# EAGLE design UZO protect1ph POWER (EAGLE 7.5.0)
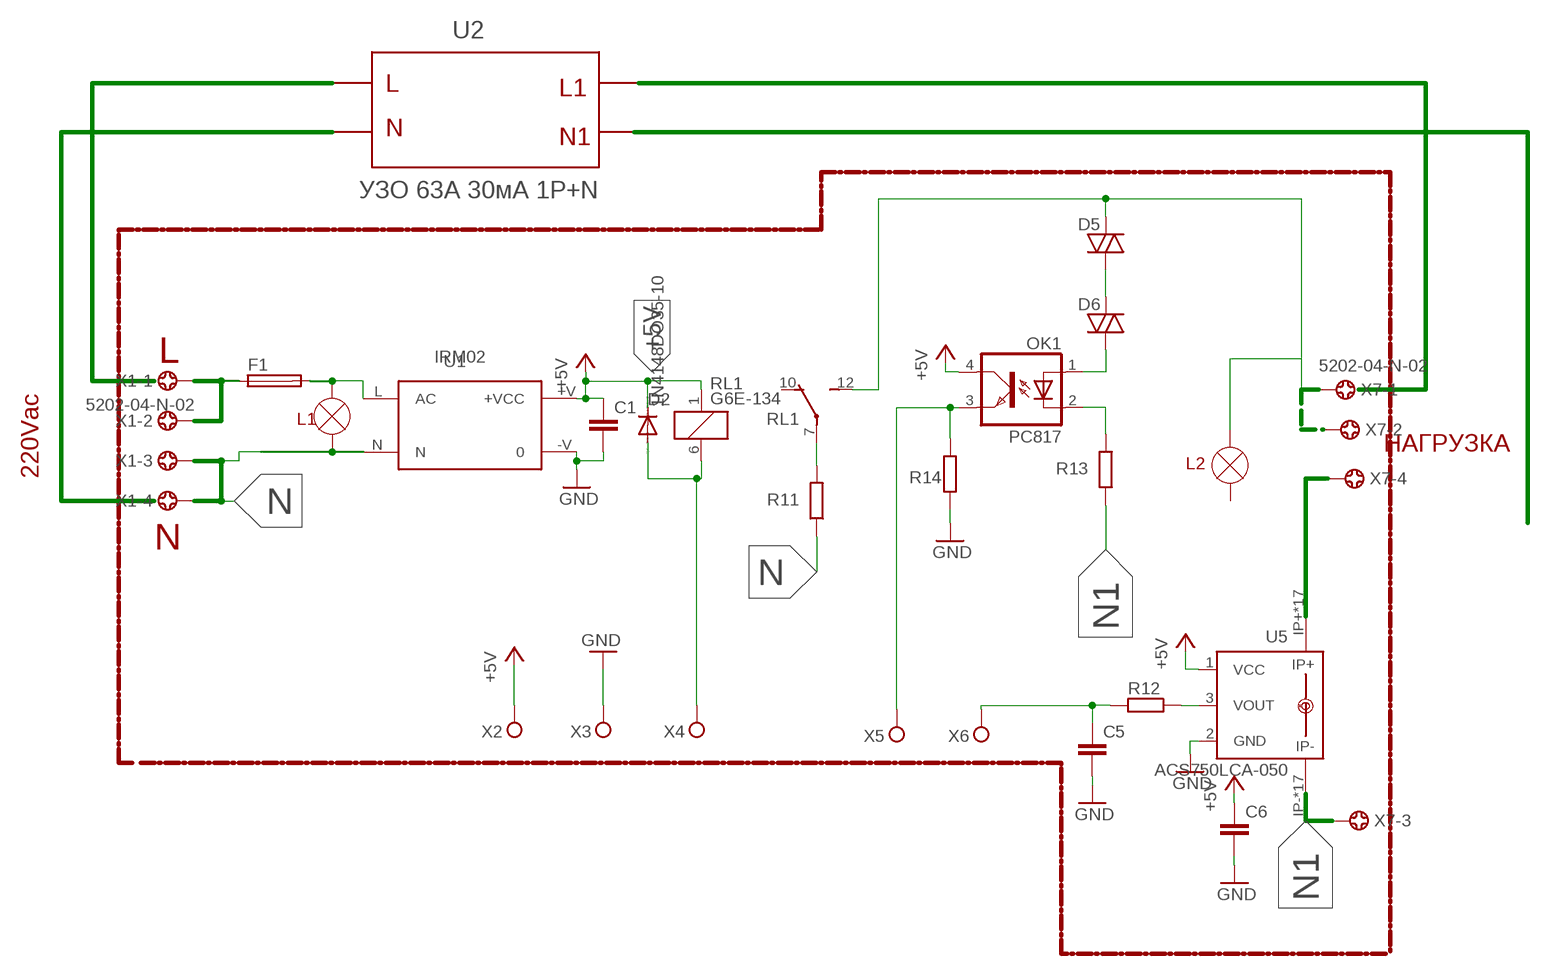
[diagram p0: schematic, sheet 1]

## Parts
C1  C-EUC1206  [C1206]
C5  C-EUC1206  [C1206]
C6  C-EUC1206  [C1206]
D2  1N4148DO35-10  [DO35-10]
D5  DIAC-DO35-10  [DO35-10]
D6  DIAC-DO35-10  [DO35-10]
F1  FUSEGSH15 1A 5x20mm  FUSEGSH15  [GSH15]
OK1  PC817  [DIL04]
R11  R-EU_0817/22  [P0817/22]
R12  R-EU_R1206  [R1206]
R13  R-EU_0817/22  [P0817/22]
R14  R-EU_R1206  [R1206]
RL1  G6E-134  [G6E]
U1  IRM02  [IRM02]
U5  ACS750LCA-050  [ACS75050]
X1  5202-04-N-02  [5202-04-N-02]
X2  TPPAD1-17  [P1-17]
X3  TPPAD1-17  [P1-17]
X4  TPPAD1-17  [P1-17]
X5  TPPAD1-17  [P1-17]
X6  TPPAD1-17  [P1-17]
X7  5202-04-N-02  [5202-04-N-02]

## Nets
+5V: C1.1 C6.1 D2.C OK1.4(COL) RL1.1 U1.+V(+VCC) U5.1(VCC) X2.TP
GND: C1.2 C5.2 C6.2 R14.1 U1.-V U5.2(GND) X3.TP
N: R11.1 U1.N X1.3 X1.4
N1: R13.1 U5.IP- U5.IP-@2(IP-) U5.IP-@3(IP-) U5.IP-@4(IP-) U5.IP-@5(IP-) U5.IP-@6(IP-) U5.IP-@7(IP-) U5.IP-@8(IP-) U5.IP-@9(IP-) U5.IP-@10(IP-) U5.IP-@11(IP-) U5.IP-@12(IP-) U5.IP-@13(IP-) U5.IP-@14(IP-) U5.IP-@15(IP-) U5.IP-@16(IP-) U5.IP-@17(IP-) X7.3
N$1: F1.1 X1.1 X1.2
N$2: R11.2 RL1.7(P)
N$3: F1.2 U1.L(AC)
N$4: D2.A RL1.6 X4.TP
N$5: U5.IP+ U5.IP+@2(IP+) U5.IP+@3(IP+) U5.IP+@4(IP+) U5.IP+@5(IP+) U5.IP+@6(IP+) U5.IP+@7(IP+) U5.IP+@8(IP+) U5.IP+@9(IP+) U5.IP+@10(IP+) U5.IP+@11(IP+) U5.IP+@12(IP+) U5.IP+@13(IP+) U5.IP+@14(IP+) U5.IP+@15(IP+) U5.IP+@16(IP+) U5.IP+@17(IP+) X7.4
N$8: D5.A D6.C
N$9: D6.A OK1.1(A)
N$10: OK1.2(C) R13.2
N$11: OK1.3(EMIT) R14.2 X5.TP
N$12: R12.1 U5.3(VOUT)
N$13: C5.1 R12.2 X6.TP
N$17: D5.C RL1.12(S) X7.1 X7.2
Unconnected: RL1.10(O)

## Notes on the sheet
- U2
- L | L1
- N
- N1
- УЗО 63А 30мА 1Р+N
- L
- L1
- НАГРУЗКА
- L2
- 220Vac
- N

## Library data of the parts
C1 C5 C6 = rcl:C-EU: CAPACITOR, European symbol
D2 = diode:1N4148: DIODE
D5 D6 = diode:DIAC-: DIAC
F1 = fuse:FUSE: Fuse; OC_FARNELL: unknown; OC_NEWARK: unknown
OK1 = optocoupler:PC817: SHARP OPTO COUPLER; MPN: PC817X4J000F; OC_FARNELL: 9707727; OC_NEWARK: 97K7059
R11-R14 = rcl:R-EU_: RESISTOR, European symbol
RL1 = relay:G6E-134
U1 = acdc:IRM02: 2W Single Output ACDC converter
U5 = allegro:ACS750*CA-050: Current Sensor display layer 49 Reference in BRD and place VIAs on circles Source: www.allegromicro.com/datafile/0750-050.pdf; MF: ALLEGRO MICROSYSTEMS, INC.; MPN: ACS750LCA-050; OC_FARNELL: 1457176; OC_NEWARK: 61H4464
X1 X7 = con-ebyelectro:5202-04-N-02: Barrier Blocks Sreies 5202 Source: http://www.ebyelectro.com/PDF/5202-XX-N-02.pdf; OC_FARNELL: unknown; OC_NEWARK: unknown
X2-X6 = testpad:TP: Test pad

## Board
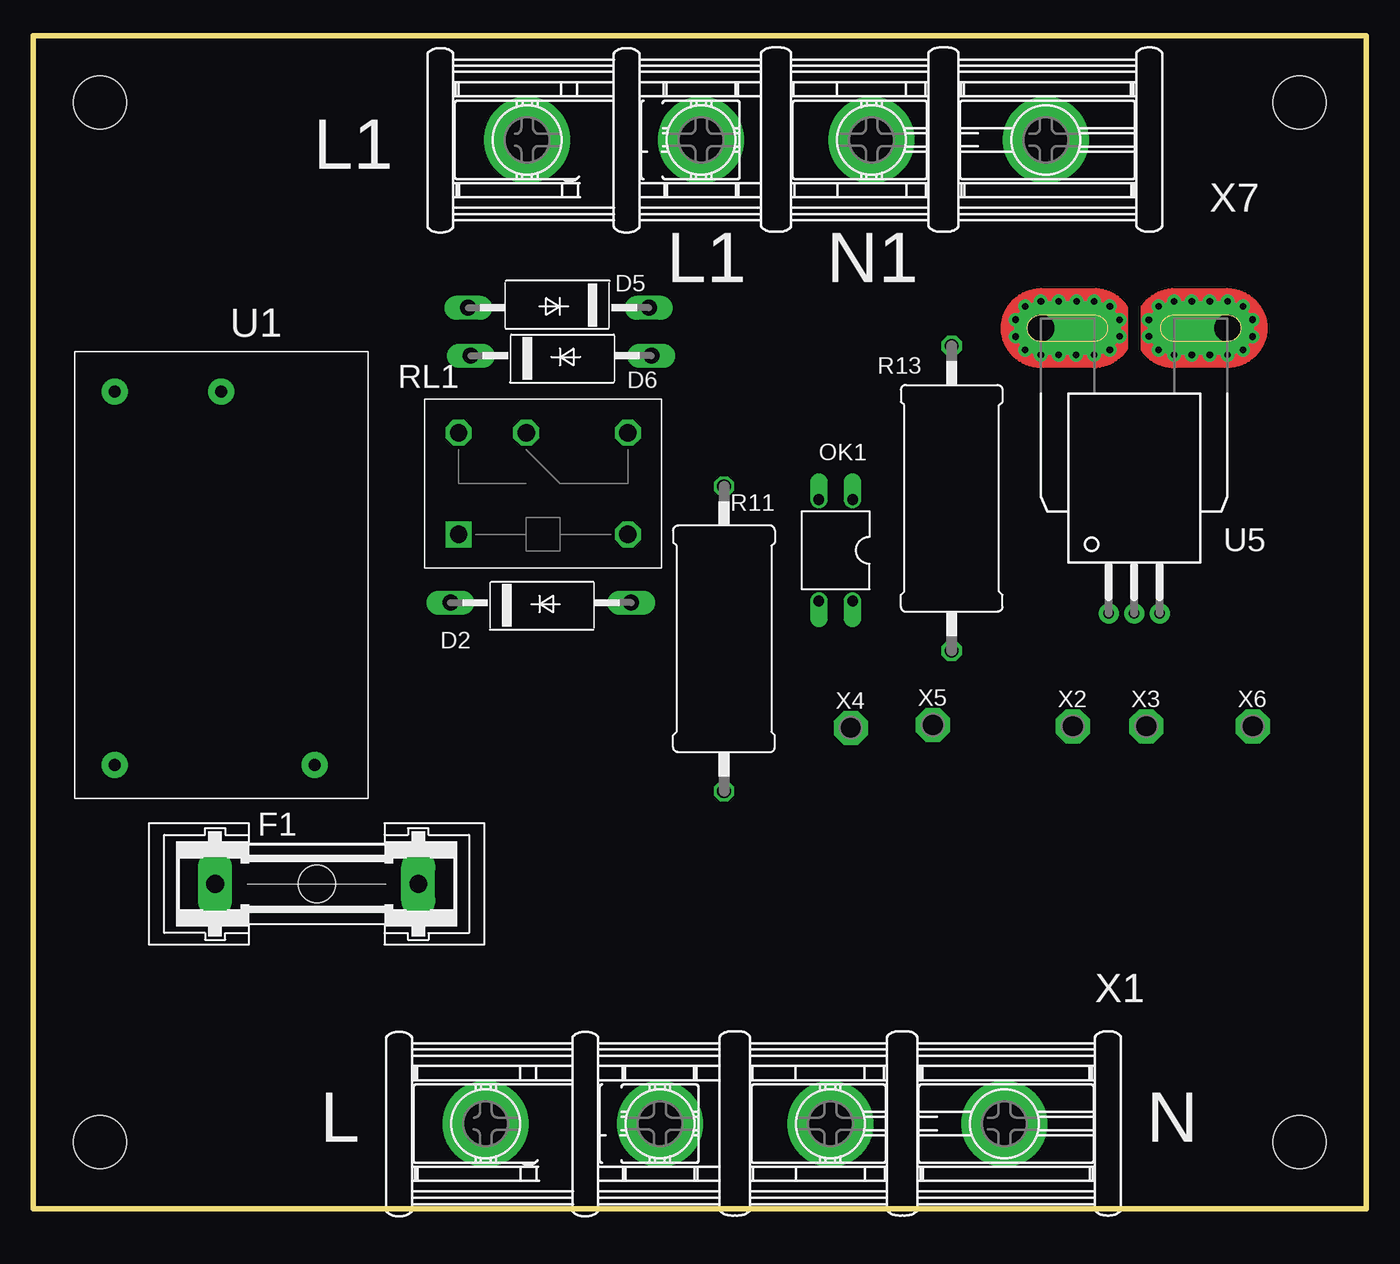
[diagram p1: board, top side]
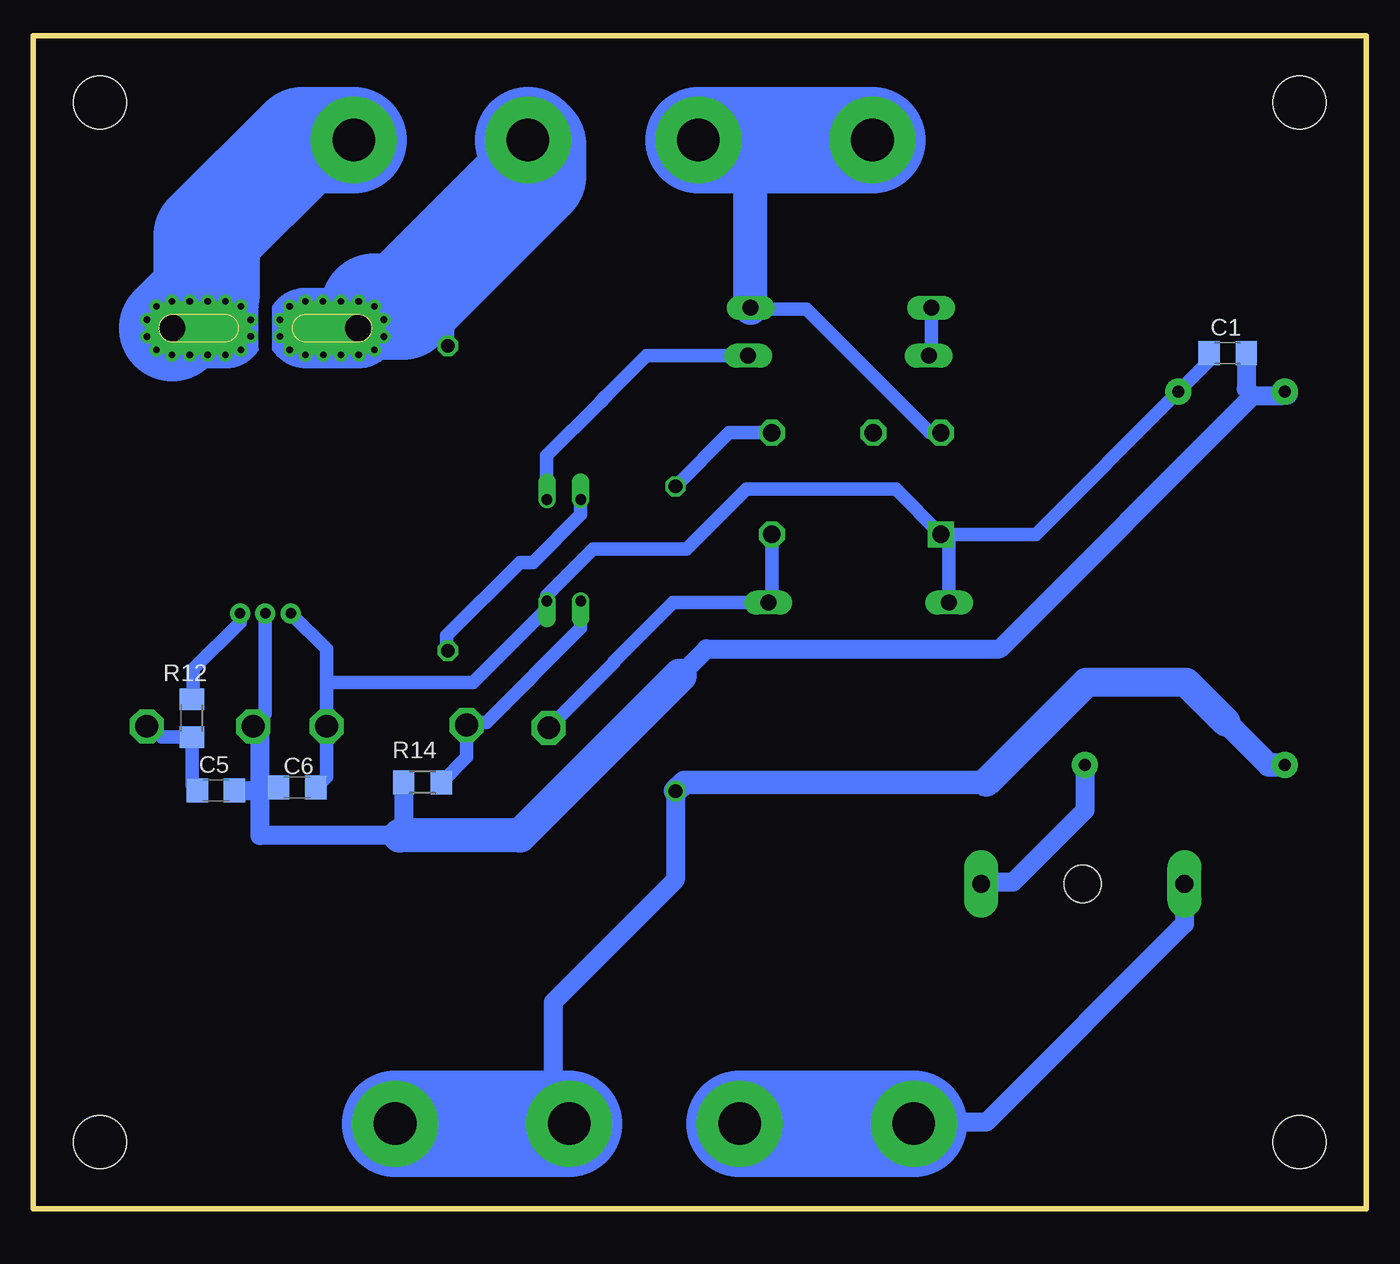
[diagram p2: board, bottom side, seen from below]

Size 100 x 88 mm. Coordinates in mm from the lower left corner, seen from the top.
Outline: 0,0 100,0 100,88 0,88 0,0
Copper layers (1*16): Top 0.035mm / dielectric 1.5mm / Bottom 0.035mm
Design rules "default *": minimum track width 10mil, minimum drill 10mil, track to track 8mil, track to pad 8mil, pad to pad 8mil, via to via 8mil, smd to smd 8mil, copper to edge 40mil, drill to drill 8mil, minimum pad ring 10mil, minimum via ring 8mil, stop-mask expansion 4mil, vias tented up to drill 0mil, thermal gap 10mil
Holes 4 mm at 5,5 95,5 95,83 5,83

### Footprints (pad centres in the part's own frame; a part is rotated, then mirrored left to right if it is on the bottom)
C1206 = smd 1.6 x 1.8: 1 -1.4,0; 2 1.4,0
DO35-10 = drill 1.2 long: A 8.18,0; C -5.38,0
GSH15 = drill 1.321 pad 2.54 long: 1 -7.62,0; 2 7.62,0 | hole 2.794: 0,0
DIL04 = drill 0.813 offset: 1 -1.27,-3.81; 2 1.27,-3.81; 3 1.27,3.81; 4 -1.27,3.81
P0817/22 = drill 1.016 octagon: 1 -11.43,0; 2 11.43,0
R1206 = smd 1.6 x 1.803: 1 -1.422,0; 2 1.422,0
G6E = drill 1.3 square: 1 0,0 | drill 1.3 octagon: 6 12.7,0; 7 12.7,7.62; 10 5.08,7.62; 12 0,7.62
IRM02 = drill 0.9 pad 1.93: +V 30.5,-11; -V 30.5,-3; L 2.5,-18; N 2.5,-3
ACS75050 = drill 0.8 pad 1.5: 1 -1.91,-21.4; 2 0,-21.4; 3 1.91,-21.4 | drill 2 pad 4 offset: IP+ 7,0; IP- -7,0 | drill 0.5 pad 0.9: IP+@2 8.89,-0.635; IP+@3 8.89,0.635; IP+@4 8.175,1.625; IP+@5 7,2; IP+@6 5.675,2; IP+@7 4.325,2; IP+@8 3,2; IP+@9 1.825,1.625; IP+@10 1.1,0.625; IP+@11 1.1,-0.625; IP+@12 1.825,-1.625; IP+@13 3,-2; IP+@14 4.325,-2; IP+@15 5.675,-2; IP+@16 7,-2; IP+@17 8.175,-1.625; IP-@2 -8.89,-0.635; IP-@3 -8.89,0.635; IP-@4 -8.175,1.625; IP-@5 -7,2; IP-@6 -5.675,2; IP-@7 -4.325,2; IP-@8 -3,2; IP-@9 -1.825,1.625; IP-@10 -1.1,0.625; IP-@11 -1.1,-0.625; IP-@12 -1.825,-1.625; IP-@13 -3,-2; IP-@14 -4.35,-2; IP-@15 -5.675,-2; IP-@16 -7,-2; IP-@17 -8.175,-1.625
5202-04-N-02 = drill 3.2 pad 6.452: 1 -14.875,0; 2 -1.815,0; 3 10.975,0; 4 24.035,0
P1-17 = drill 1.702 pad 2.54 octagon: TP 0,0

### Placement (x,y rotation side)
C1  10.4,64.21 0 bottom
C5  86.3,31.4 0 bottom
C6  80.2,31.6 180 bottom
D2  36.68,45.47 0 top
D5  40.8,67.6 180 top
D6  38.2,64 0 top
F1  21.26,24.37 0 top
OK1  60.2,49.4 180 top
R11  51.82,42.76 90 top
R12  88.1,36.8 270 bottom
R13  68.9,53.3 270 top
R14  70.8,32 0 bottom
RL1  31.9,50.6 0 top
U1  3.1,30.8 90 top
U5  82.59,66.07 0 top
X1  48.82,6.38 0 top
X2  78,36.2 0 top
X3  83.5,36.2 0 top
X4  61.33,36.08 0 top
X5  67.5,36.3 0 top
X6  91.5,36.2 0 top
X7  51.92,80.19 0 top

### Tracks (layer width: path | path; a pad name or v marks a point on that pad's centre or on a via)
+5V
  Bottom 1.016: 61.5,45.62 OK1.4 | 78,39.5 X2.TP 78,32.4 C6.1 | OK1.4 61.47,45.03 67,39.5 78,39.5 | 78,39.5 78,41.99 U5.1 | OK1.4 61.47,46.03 58,49.5 51,49.5 46.5,54 35.3,54 RL1.1 | C1.1 11.8,63.6 U1.+V 24.8,50.6 RL1.1 | D2.C 31.3,50 RL1.1
GND
  Bottom 1.016: U5.2 82.59,37.11 X3.TP | 72.5,28 73,28 | C1.2
  Bottom 1.422: 51.5,40 49.5,42 27.5,42 8.5,61 | 8.5,61 6.4,61 U1.-V | C1.2 9,61.5 8.5,61 | 73,28 83,28 83,31.5 | 83,31.5 83,35.7 X3.TP | C6.2 82.9,31.6 83,31.5 | C5.2 83.1,31.4 83,31.5 | R14.1 72.22,28.28 72.5,28
  Bottom 1.778: 6,61.2 U1.-V
  Bottom 2.54: 51.5,40 63.5,28 72.5,28
N
  Bottom 1.422: R11.1 51.82,24.68 61,15.5 61,8.5 60.5,8 60.5,7.08 X1.3
  Bottom 1.778: U1.N 7.3,33.3 10.5,36.5 | 28.5,32 51.15,32 R11.1
  Bottom 2.184: 10.5,36.5 13.5,39.5 21,39.5 28.5,32
  Bottom 8: X1.4 X1.3
N1
  Bottom 1.016: R13.1 68.9,65.9 71.5,68.5
  Bottom 8: U5.IP-@4 72.31,67.69 71.5,68.5 62.5,77.5 62.5,79.8 X7.3
N$1
  Bottom 1.422: F1.1 13.64,21.36 28.5,6.5 33.83,6.5 X1.1
  Bottom 8: X1.2 X1.1
N$2
  Bottom 1.016: RL1.7 47.79,58.22 R11.2
N$3
  Bottom 1.422: U1.L 21.1,29.9 26.5,24.5 28.75,24.5 F1.2
N$4
  Bottom 1.016: X4.TP 56.44,40.97 56.44,41.06 52,45.5 44.89,45.5 D2.A 44.6,45.73 RL1.6
N$5
  Bottom 8: X7.4 79.81,80.19 87,73 87,68.66 U5.IP+
N$8
  Bottom 1.016: D5.A 32.62,64.2 D6.C
N$9
  Bottom 1.016: OK1.1 61.5,53.24 61.5,56.5 57.5,60.5 57,61 54,64 D6.A
N$10
  Bottom 1.016: OK1.2 58.93,52.07 62.5,48.5 63.5,48.5 69,43 69,41.97 R13.2
N$11
  Bottom 1.016: 59,45.66 OK1.3 58.93,43.57 66,36.5 67.3,36.5 X5.TP 67.5,33.88 R14.2
N$12
  Bottom 1.016: U5.3 84.5,44 88,40.5 88,38.32 R12.1
N$13
  Bottom 1.016: X6.TP 91.3,36 91,36 90.38,35.38 R12.2 88.1,31.8 C5.1
N$17
  Bottom 1.016: 46.68,77.37 49.5,80.19 | RL1.12 32.72,58.22 42,67.5 46.08,67.5 D5.C
  Bottom 2.54: D5.C 46.18,76.87 46.68,77.37
  Bottom 8: X7.1 49.5,80.19 X7.2

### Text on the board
tPlace: L1 | L1 | N1 | L | N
